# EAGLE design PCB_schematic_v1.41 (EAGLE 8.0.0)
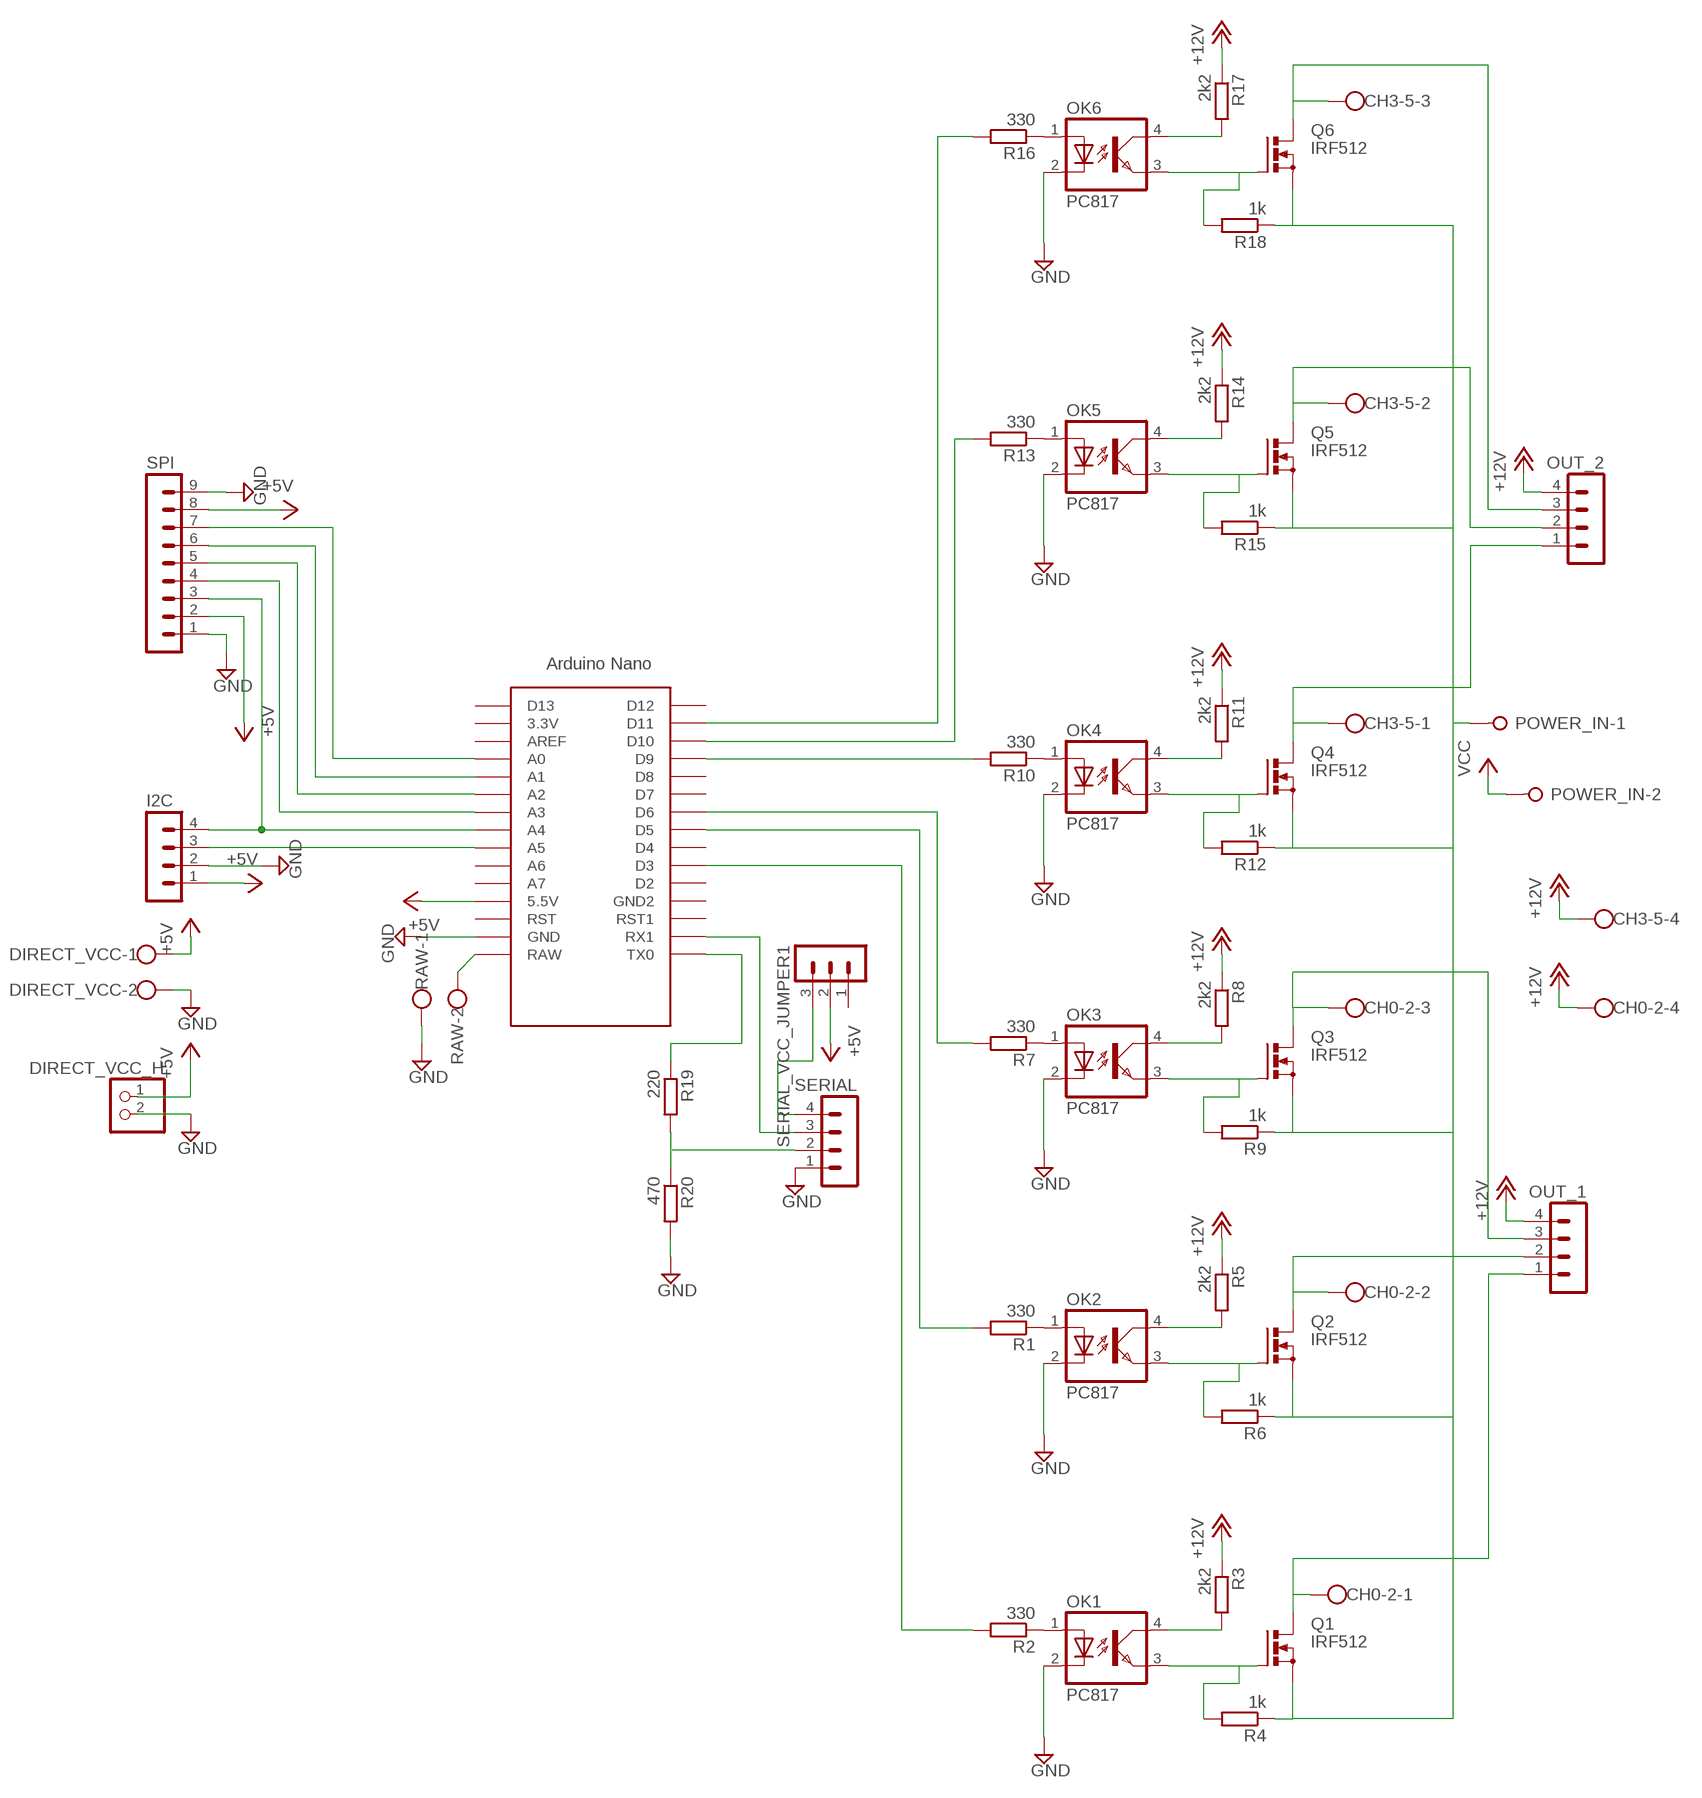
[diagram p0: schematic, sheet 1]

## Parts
CH0-2  W237-4  [W237-4]
CH3-5  W237-4  [W237-4]
DIRECT_VCC  W237-102  [W237-102]
DIRECT_VCC_H  PINHD-1X2  [1X02]
I2C  MA04-1  [MA04-1]
OK1  PC817  [DIL04]
OK2  PC817  [DIL04]
OK3  PC817  [DIL04]
OK4  PC817  [DIL04]
OK5  PC817  [DIL04]
OK6  PC817  [DIL04]
OUT_1  MA04-1  [MA04-1]
OUT_2  MA04-1  [MA04-1]
POWER_IN  W237-02P  [W237-132]
Q1  IRF512  [TO220BV]
Q2  IRF512  [TO220BV]
Q3  IRF512  [TO220BV]
Q4  IRF512  [TO220BV]
Q5  IRF512  [TO220BV]
Q6  IRF512  [TO220BV]
R1  330  R-EU_0207/10  [0207/10]
R2  330  R-EU_0207/10  [0207/10]
R3  2k2  R-EU_0207/10  [0207/10]
R4  1k  R-EU_0207/10  [0207/10]
R5  2k2  R-EU_0207/10  [0207/10]
R6  1k  R-EU_0207/10  [0207/10]
R7  330  R-EU_0207/10  [0207/10]
R8  2k2  R-EU_0207/10  [0207/10]
R9  1k  R-EU_0207/10  [0207/10]
R10  330  R-EU_0207/10  [0207/10]
R11  2k2  R-EU_0207/10  [0207/10]
R12  1k  R-EU_0207/10  [0207/10]
R13  330  R-EU_0207/10  [0207/10]
R14  2k2  R-EU_0207/10  [0207/10]
R15  1k  R-EU_0207/10  [0207/10]
R16  330  R-EU_0207/10  [0207/10]
R17  2k2  R-EU_0207/10  [0207/10]
R18  1k  R-EU_0207/10  [0207/10]
R19  220  R-EU_0207/10  [0207/10]
R20  470  R-EU_0207/10  [0207/10]
RAW  W237-102  [W237-102]
SERIAL  MA04-1  [MA04-1]
SERIAL_VCC_JUMPER1  MA03-1  [MA03-1]
SPI  MA09-1  [MA09-1]
U$1  NANO  [NANO]

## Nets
+5V: DIRECT_VCC.1 DIRECT_VCC_H.1 I2C.1 SERIAL_VCC_JUMPER1.2 SPI.2 SPI.8 U$1.5V(5.5V)
+12V: CH0-2.4 CH3-5.4 OUT_1.4 OUT_2.4 R3.1 R5.1 R8.1 R11.1 R14.1 R17.1
CS: SPI.7 U$1.A0
D1: SPI.4 U$1.A3
DC: SPI.6 U$1.A1
EXT_GND: POWER_IN.1 Q1.S Q2.S Q3.S Q4.S Q5.S Q6.S R4.1 R6.1 R9.1 R12.1 R15.1 R18.1
EXT_VCC_12V: POWER_IN.2 ; supply symbol labelled VCC
FET0_GATE: OK1.3(EMIT) Q1.G R4.2
FET0_GATE1: OK2.3(EMIT) Q2.G R6.2
FET0_GATE2: OK3.3(EMIT) Q3.G R9.2
FET0_GATE3: OK4.3(EMIT) Q4.G R12.2
FET0_GATE4: OK5.3(EMIT) Q5.G R15.2
FET0_GATE5: OK6.3(EMIT) Q6.G R18.2
GND: DIRECT_VCC.2 DIRECT_VCC_H.2 I2C.2 OK1.2(C) OK2.2(C) OK3.2(C) OK4.2(C) OK5.2(C) OK6.2(C) R20.2 RAW.1 SERIAL.1 SPI.1 SPI.9 U$1.GND
IC_PWM_OUT_0: R2.2 U$1.D3
IC_PWM_OUT_0_BASE: OK1.1(A) R2.1
IC_PWM_OUT_0_BASE1: OK2.1(A) R1.1
IC_PWM_OUT_0_BASE2: OK3.1(A) R7.1
IC_PWM_OUT_0_BASE3: OK4.1(A) R10.1
IC_PWM_OUT_0_BASE4: OK5.1(A) R13.1
IC_PWM_OUT_0_BASE5: OK6.1(A) R16.1
IC_PWM_OUT_1: R1.2 U$1.D5
IC_PWM_OUT_2: R7.2 U$1.D6
IC_PWM_OUT_3: R10.2 U$1.D9
IC_PWM_OUT_4: R13.2 U$1.D10
IC_PWM_OUT_5: R16.2 U$1.D11
N$1: OK1.4(COL) R3.2
N$3: OK2.4(COL) R5.2
N$5: OK3.4(COL) R8.2
N$7: OK4.4(COL) R11.2
N$9: OK5.4(COL) R14.2
N$11: OK6.4(COL) R17.2
OLED_RES: SPI.5 U$1.A2
OUTPUT_0: CH0-2.1 OUT_1.1 Q1.D
OUTPUT_1: CH0-2.2 OUT_1.2 Q2.D
OUTPUT_2: CH0-2.3 OUT_1.3 Q3.D
OUTPUT_3: CH3-5.1 OUT_2.1 Q4.D
OUTPUT_4: CH3-5.2 OUT_2.2 Q5.D
OUTPUT_5: CH3-5.3 OUT_2.3 Q6.D
RAW_INPUT: RAW.2 U$1.RAW
RX: SERIAL.3 U$1.RX1
SCL: I2C.3 U$1.A5
SDA_/_D0: I2C.4 SPI.3 U$1.A4
SERIAL_VCC: SERIAL.4 SERIAL_VCC_JUMPER1.3
TX_3,3V: R19.2 R20.1 SERIAL.2
TX_5V: R19.1 U$1.TX0
Unconnected: SERIAL_VCC_JUMPER1.1 U$1.3.3V U$1.A6 U$1.A7 U$1.AREF U$1.D2 U$1.D4 U$1.D7 U$1.D8 U$1.D12 U$1.D13 U$1.GND1(GND2) U$1.ICSP1 U$1.ICSP2 U$1.ICSP3 U$1.ICSP4 U$1.ICSP5 U$1.ICSP6 U$1.RST U$1.RST1

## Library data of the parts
CH0-2 CH3-5 = con-wago-500:W237-4: WAGO SCREW CLAMP; OC_FARNELL: unknown; OC_NEWARK: unknown
DIRECT_VCC RAW = con-wago-500:W237-102: WAGO SCREW CLAMP; MPN: 237-102; OC_FARNELL: unknown; OC_NEWARK: 70K9898
DIRECT_VCC_H = pinhead:PINHD-1X2: PIN HEADER
I2C OUT_1 OUT_2 SERIAL = con-lstb:MA04-1: PIN HEADER; OC_FARNELL: unknown; OC_NEWARK: unknown
OK1-OK6 = optocoupler:PC817: SHARP OPTO COUPLER; MPN: PC817X4J000F; OC_FARNELL: 9707727; OC_NEWARK: 97K7059
POWER_IN = con-wago-508:W237-02P: WAGO SREW CLAMP; OC_FARNELL: unknown; OC_NEWARK: unknown
Q1-Q6 = transistor-power:IRF512: N-CHANNEL MOS FET
R1-R20 = rcl:R-EU_: RESISTOR, European symbol
SERIAL_VCC_JUMPER1 = con-lstb:MA03-1: PIN HEADER; OC_FARNELL: unknown; OC_NEWARK: unknown
SPI = con-lstb:MA09-1: PIN HEADER; OC_FARNELL: unknown; OC_NEWARK: unknown
U$1 = Arduino-clone:NANO: Arduino Nano

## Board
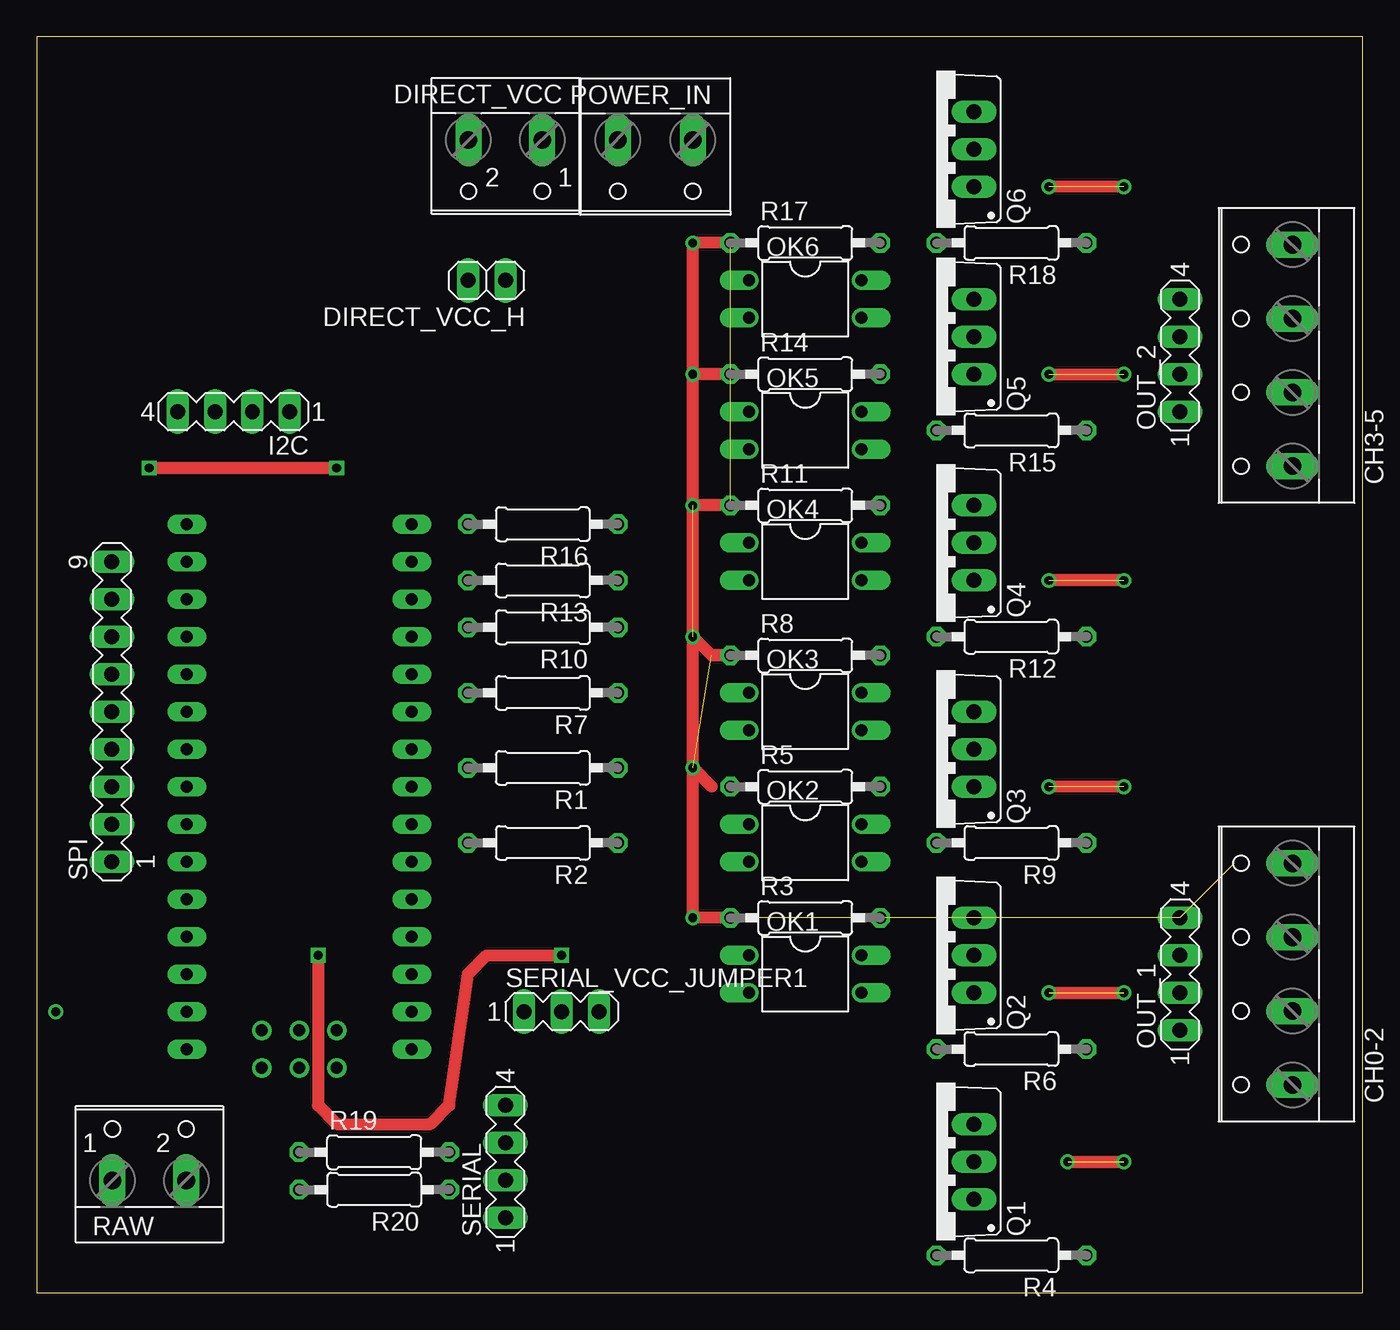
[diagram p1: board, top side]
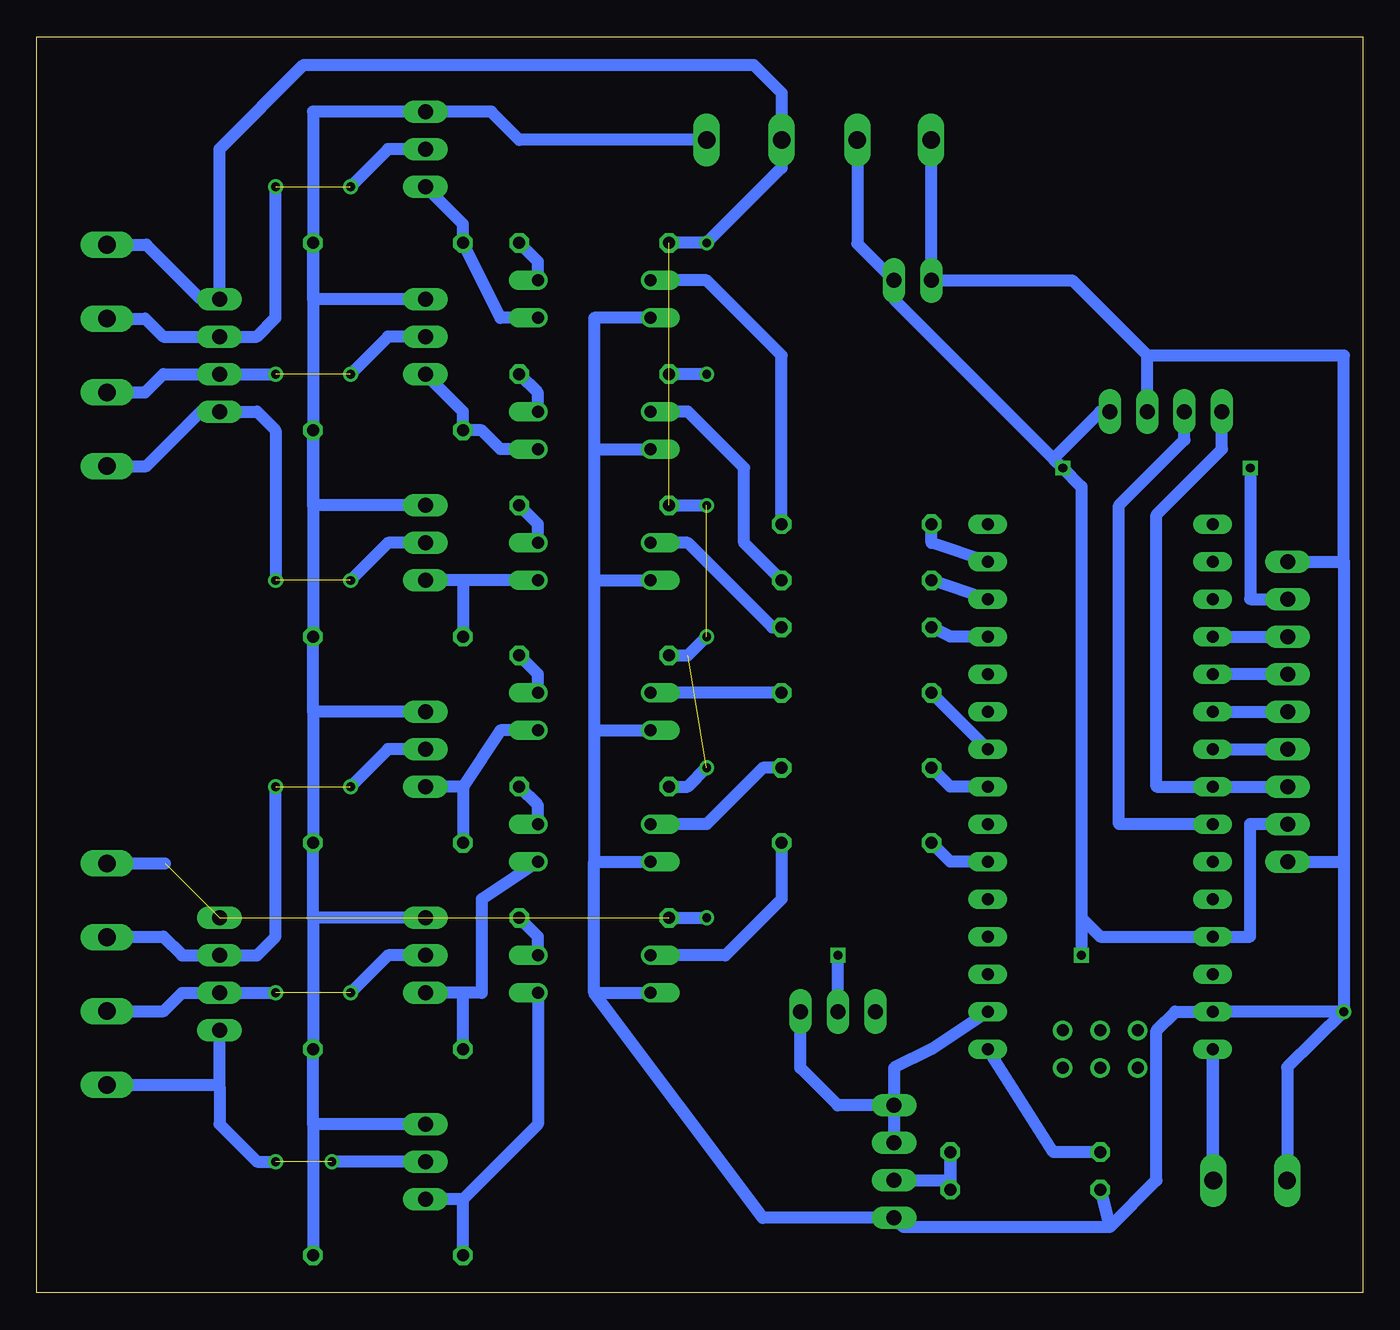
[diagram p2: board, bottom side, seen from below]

Size 89.84 x 85.08 mm. Coordinates in mm from the lower left corner, seen from the top.
Outline: 0,0 89.84,0 89.84,85.08 0,85.08 0,0
Copper layers (1*16): Top 0.035mm / dielectric 1.5mm / Bottom 0.035mm
Design rules "default": minimum track width 10mil, minimum drill 24mil, track to track 8mil, track to pad 8mil, pad to pad 8mil, via to via 8mil, smd to smd 8mil, copper to edge 40mil, drill to drill 8mil, minimum pad ring 10mil, minimum via ring 8mil, stop-mask expansion 4mil, vias tented up to drill 0mil, thermal gap 10mil

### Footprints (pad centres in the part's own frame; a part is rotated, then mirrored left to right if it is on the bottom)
W237-4 = drill 1.194 long: 1 -7.5,-1.27; 2 -2.5,-1.27; 3 2.5,-1.27; 4 7.5,-1.27
W237-102 = drill 1.194 long: 1 -2.5,-1.27; 2 2.5,-1.27
1X02 = drill 1.016 long: 1 -1.27,0; 2 1.27,0
MA04-1 = drill 1.016 long: 1 -3.81,0; 2 -1.27,0; 3 1.27,0; 4 3.81,0
DIL04 = drill 0.813 offset: 1 -1.27,-3.81; 2 1.27,-3.81; 3 1.27,3.81; 4 -1.27,3.81
W237-132 = drill 1.194 long: 1 -2.54,-0.635; 2 2.54,-0.635
TO220BV = drill 1.016 long: D 0,-2.54; G -2.54,-2.54; S 2.54,-2.54
0207/10 = drill 0.813 octagon: 1 -5.08,0; 2 5.08,0
MA03-1 = drill 1.016 long: 1 -2.54,0; 2 0,0; 3 2.54,0
MA09-1 = drill 1.016 long: 1 -10.16,0; 2 -7.62,0; 3 -5.08,0; 4 -2.54,0; 5 0,0; 6 2.54,0; 7 5.08,0; 8 7.62,0; 9 10.16,0
NANO = drill 0.8 long: 3.3V -10.16,24.13; 5V -10.16,-1.27; A0 -10.16,19.05; A1 -10.16,16.51; A2 -10.16,13.97; A3 -10.16,11.43; A4 -10.16,8.89; A5 -10.16,6.35; A6 -10.16,3.81; A7 -10.16,1.27; AREF -10.16,21.59; D2 5.08,1.27; D3 5.08,3.81; D4 5.08,6.35; D5 5.08,8.89; D6 5.08,11.43; D7 5.08,13.97; D8 5.08,16.51; D9 5.08,19.05; D10 5.08,21.59; D11 5.08,24.13; D12 5.08,26.67; D13 -10.16,26.67; GND -10.16,-6.35; GND1 5.08,-1.27; RAW -10.16,-8.89; RST -10.16,-3.81; RST1 5.08,-3.81; RX1 5.08,-6.35; TX0 5.08,-8.89 | drill 0.8: ICSP1 -5.08,-10.16; ICSP2 -5.08,-7.62; ICSP3 -2.54,-10.16; ICSP4 -2.54,-7.62; ICSP5 0,-10.16; ICSP6 0,-7.62

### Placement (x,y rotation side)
CH0-2  83.82,21.59 90 top
CH3-5  83.82,63.5 90 top
DIRECT_VCC  31.75,76.83 180 top
DIRECT_VCC_H  30.48,68.58 180 top
I2C  13.34,59.69 180 top
OK1  52.07,21.59 270 top
OK2  52.07,30.48 270 top
OK3  52.07,39.37 270 top
OK4  52.07,49.53 270 top
OK5  52.07,58.42 270 top
OK6  52.07,67.31 270 top
OUT_1  77.47,21.59 90 top
OUT_2  77.47,63.5 90 top
POWER_IN  41.91,77.47 180 top
Q1  60.96,8.89 90 top
Q2  60.96,22.86 90 top
Q3  60.96,36.83 90 top
Q4  60.96,50.8 90 top
Q5  60.96,64.77 90 top
Q6  60.96,77.47 90 top
R1  34.29,35.56 180 top
R2  34.29,30.48 180 top
R3  52.07,25.4 0 top
R4  66.04,2.54 180 top
R5  52.07,34.29 0 top
R6  66.04,16.51 180 top
R7  34.29,40.64 180 top
R8  52.07,43.18 0 top
R9  66.04,30.48 180 top
R10  34.29,45.09 180 top
R11  52.07,53.34 0 top
R12  66.04,44.45 180 top
R13  34.29,48.26 180 top
R14  52.07,62.23 0 top
R15  66.04,58.42 180 top
R16  34.29,52.07 180 top
R17  52.07,71.12 0 top
R18  66.04,71.12 180 top
R19  22.86,9.53 0 top
R20  22.86,6.99 180 top
RAW  7.62,8.89 0 top
SERIAL  31.75,8.89 90 top
SERIAL_VCC_JUMPER1  35.56,19.05 0 top
SPI  5.08,39.37 90 top
U$1  20.32,25.4 0 top

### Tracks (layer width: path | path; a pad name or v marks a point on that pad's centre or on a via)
+5V  (via drill 0.6)
  Top 0.813: v7.62,55.88 v20.32,55.88 | v19.05,22.86 19.05,12.7 20.32,11.43 26.67,11.43 27.94,12.7 29.21,21.59 30.48,22.86 v35.56,22.86
  Bottom 0.813: DIRECT_VCC.1 34.25,71.08 DIRECT_VCC_H.1 31.75,67.31 20.95,56.52 | 19.05,25.4 19.05,54.61 v20.32,55.88 20.95,56.52 | 19.05,25.4 17.78,24.13 U$1.5V 7.62,24.13 7.62,31.75 SPI.2 | v7.62,55.88 7.62,46.99 SPI.8 | 19.05,25.4 v19.05,22.86 | SERIAL_VCC_JUMPER1.2 v35.56,22.86 | I2C.1 17.78,59.69 20.95,56.52
+12V  (7 unrouted)
  Top 0.813: R11.1 44.45,53.34 | R8.1 45.72,43.18 44.45,44.45 | R17.1 44.45,71.12 | R14.1 44.45,62.23 | 45.72,34.29 44.45,35.56 44.45,25.4 R3.1
  Bottom 0.813: R11.1 44.45,53.34 | R8.1 45.72,43.18 44.45,44.45 | R5.1 45.72,34.29 44.45,35.56 | CH0-2.4 81.16,29.09 | R3.1 44.45,25.4 | CH3-5.4 82.43,71 78.74,67.31 OUT_2.4 77.47,77.47 71.75,83.19 41.27,83.19 39.37,81.28 39.37,76.2 44.45,71.12 R17.1
CS
  Bottom 0.813: U$1.A0 SPI.7
D1
  Bottom 0.813: U$1.A3 SPI.4
DC
  Bottom 0.813: SPI.6 U$1.A1
EXT_GND
  Bottom 0.813: 71.12,11.43 R4.1 | 71.12,11.43 R6.1 71.12,25.4 | 71.12,25.4 R9.1 71.12,39.37 | 71.12,39.37 R12.1 | 71.12,53.34 R15.1 71.12,67.31 | 71.12,53.34 R12.1 | 71.12,67.31 R18.1 | R18.1 71.12,80.01 Q6.S 59.05,80.01 57.15,78.11 POWER_IN.1 | Q5.S 71.12,67.31 | Q4.S 71.12,53.34 | Q2.S 71.12,25.4 | Q1.S 71.12,11.43 | R18.1 R12.1 | Q3.S 71.12,39.37
EXT_VCC_12V
  Bottom 0.813: POWER_IN.2 39.37,76.2 44.45,71.12
FET0_GATE
  Bottom 0.813: R4.2 60.96,6.35 | OK1.3 55.88,11.43 60.96,6.35 | 60.96,6.35 Q1.G
FET0_GATE1
  Bottom 0.813: R6.2 60.96,20.32 | OK2.3 59.69,26.67 59.69,20.32 60.96,20.32 | 60.96,20.32 Q2.G
FET0_GATE2
  Bottom 0.813: 60.96,34.29 Q3.G | OK3.3 58.42,38.1 60.96,34.29 | 60.96,34.29 R9.2
FET0_GATE3
  Bottom 0.813: 60.96,48.26 R12.2 | 60.96,48.26 Q4.G | OK4.3 60.96,48.26
FET0_GATE4
  Bottom 0.813: Q5.G 60.96,59.69 R15.2 59.69,58.42 58.42,57.15 OK5.3
FET0_GATE5
  Bottom 0.813: Q6.G 60.96,72.39 R18.2 58.42,66.04 OK6.3
GND  (via drill 0.6)
  Bottom 0.813: OK6.2 52.07,66.04 52.07,57.15 | 52.07,57.15 OK5.2 | 52.07,57.15 52.07,48.26 | 52.07,48.26 OK4.2 | 52.07,48.26 52.07,38.1 | 52.07,38.1 OK3.2 | 52.07,38.1 52.07,29.21 | 52.07,29.21 OK2.2 | 52.07,20.32 52.07,29.21 | 52.07,20.32 OK1.2 | 52.07,20.32 40.64,5.08 SERIAL.1 31.11,4.45 17.14,4.45 | R20.2 17.14,4.45 | 17.14,4.45 13.97,7.62 13.97,17.78 12.7,19.05 U$1.GND v1.27,19.05 | 14.61,63.5 1.27,63.5 1.27,49.53 | 1.27,49.53 1.27,29.21 | 1.27,29.21 v1.27,19.05 | v1.27,19.05 5.12,15.28 RAW.1 | SPI.1 1.27,29.21 | SPI.9 1.27,49.53 | 14.61,63.5 19.68,68.58 DIRECT_VCC_H.2 29.25,68.62 DIRECT_VCC.2 | I2C.2 14.61,63.5
IC_PWM_OUT_0
  Bottom 0.813: U$1.D3 27.94,29.21 R2.2
IC_PWM_OUT_0_BASE
  Bottom 0.813: R2.1 39.37,26.67 43.18,22.86 OK1.1
IC_PWM_OUT_0_BASE1
  Bottom 0.813: R1.1 40.64,35.56 44.45,31.75 OK2.1
IC_PWM_OUT_0_BASE2
  Bottom 0.813: R7.1 OK3.1
IC_PWM_OUT_0_BASE3
  Bottom 0.813: R10.1 40.01,45.09 45.72,50.8 OK4.1
IC_PWM_OUT_0_BASE4
  Bottom 0.813: R13.1 41.91,50.8 41.91,55.88 45.72,59.69 OK5.1
IC_PWM_OUT_0_BASE5
  Bottom 0.813: R16.1 39.37,63.5 44.45,68.58 OK6.1
IC_PWM_OUT_1
  Bottom 0.813: U$1.D5 27.94,34.29 R1.2
IC_PWM_OUT_2
  Bottom 0.813: R7.2 U$1.D6
IC_PWM_OUT_3
  Bottom 0.813: U$1.D9 27.94,44.45 R10.2
IC_PWM_OUT_4
  Bottom 0.813: U$1.D10 R13.2
IC_PWM_OUT_5
  Bottom 0.813: U$1.D11 29.21,50.8 R16.2
N$1
  Bottom 0.813: OK1.4 55.88,24.13 R3.2
N$3
  Bottom 0.813: OK2.4 55.88,33.02 R5.2
N$5
  Bottom 0.813: OK3.4 55.88,41.91 R8.2
N$7
  Bottom 0.813: OK4.4 55.88,52.07 R11.2
N$8  (via drill 0.6)
  Top 0.813: v69.85,8.89 73.66,8.89
N$9
  Bottom 0.813: OK5.4 55.88,60.96 R14.2
N$10  (via drill 0.6)
  Top 0.813: v68.58,20.32 73.66,20.32
N$11
  Bottom 0.813: OK6.4 55.88,69.85 R17.2
N$12  (via drill 0.6)  (1 unrouted)
  other vias: 68.58,34.29
N$13  (via drill 0.6)
  other vias: 68.58,48.26
N$14  (via drill 0.6)
  Top 0.813: v68.58,62.23 v73.66,62.23
N$15  (via drill 0.6)
  other vias: 68.58,74.93
N$16  (via drill 0.6)
  Top 0.813: v73.66,74.93 68.58,74.93
N$18  (via drill 0.6)
  Top 0.813: v73.66,48.26 68.58,48.26
N$19  (via drill 0.6)
  Top 0.813: v73.66,34.29 68.58,34.29
N$20  (via drill 0.6)
  other vias: 73.66,20.32
N$21  (via drill 0.6)
  other vias: 73.66,8.89
N$22  (via drill 0.6)
  Top 0.813: v44.45,25.4 44.45,53.34
N$23  (via drill 0.6)
  Top 0.813: 46.99,43.18 45.72,43.18 44.45,44.45 v44.45,35.56
N$24  (via drill 0.6)
  other vias: 44.45,44.45
N$25  (via drill 0.6)
  other vias: 44.45,53.34
N$26  (via drill 0.6)
  Top 0.813: 44.45,53.34 v44.45,62.23 44.45,71.12
  Bottom 0.813: v44.45,62.23 46.99,62.23
N$27  (via drill 0.6)
  other vias: 44.45,71.12
OLED_RES
  Bottom 0.813: U$1.A2 SPI.5
OUTPUT_0  (1 unrouted)
  Bottom 0.813: 77.47,13.97 OUT_1.1 | 77.47,13.97 77.47,11.43 74.93,8.89 73.66,8.89 | CH0-2.1 77.59,14.09 77.47,13.97 | Q1.D 69.85,8.89
OUTPUT_1  (1 unrouted)
  Bottom 0.813: 73.66,20.32 OUT_1.2 80.01,20.32 81.24,19.09 CH0-2.2 | Q2.D 66.04,22.86 68.58,20.32
OUTPUT_2  (1 unrouted)
  Bottom 0.813: Q3.D 66.04,36.83 68.58,34.29 | CH0-2.3 85.05,24.13 81.28,24.13 80.01,22.86 OUT_1.3 74.93,22.86 73.66,24.13 73.66,34.29
OUTPUT_3  (1 unrouted)
  Bottom 0.813: Q4.D 66.04,50.8 68.58,48.26 | 73.66,48.26 73.66,58.42 74.93,59.69 OUT_2.1 78.74,59.69 82.43,56 CH3-5.1
OUTPUT_4  (1 unrouted)
  Bottom 0.813: Q5.D 66.04,64.77 68.58,62.23 | CH3-5.2 82.51,61 81.28,62.23 OUT_2.2 73.66,62.23
OUTPUT_5  (1 unrouted)
  Bottom 0.813: Q6.D 66.04,77.47 68.58,74.93 | CH3-5.3 82.51,66 81.28,64.77 OUT_2.3 74.93,64.77 73.66,66.04 73.66,74.93
RAW_INPUT
  Bottom 0.813: 10.16,7.62 U$1.RAW 10.16,7.66 RAW.2
RX
  Bottom 0.813: U$1.RX1 29.21,16.51 31.75,15.24 SERIAL.3
SCL
  Bottom 0.813: U$1.A5 16.51,31.75 16.51,53.34 12.06,57.78 I2C.3
SDA_/_D0
  Bottom 0.813: I2C.4 9.53,57.15 13.97,52.7 13.97,34.29 U$1.A4 SPI.3
SERIAL_VCC
  Bottom 0.813: SERIAL.4 35.56,12.7 38.1,15.24 SERIAL_VCC_JUMPER1.3
TX_3,3V
  Bottom 0.813: R20.1 R19.2 27.94,7.62 SERIAL.2
TX_5V
  Bottom 0.813: R19.1 20.95,9.53 U$1.TX0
